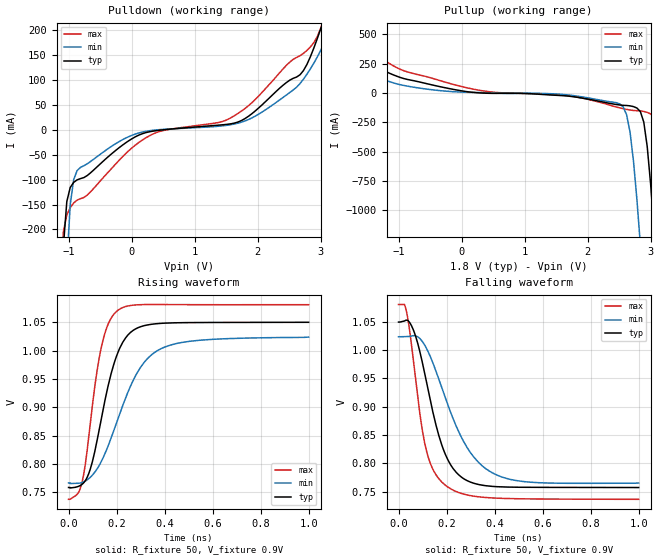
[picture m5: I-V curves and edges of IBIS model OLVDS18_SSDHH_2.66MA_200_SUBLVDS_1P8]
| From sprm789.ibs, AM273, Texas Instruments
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|   Model Cell OLVDS18_SSDHH_2.66MA_200_SUBLVDS_1P8
|OLVDS18_SSDHH_2.66MA_200_SUBLVDS_1P8
[Model]   OLVDS18_SSDHH_2.66MA_200_SUBLVDS_1P8
Model_type   Output
Polarity   Non-Inverting
Cref =  15.0001pF
Rref =  101.0000M
Vref =  0V
Vmeas =  1.08
C_comp   1.5p   1.5p   1.5p
[Temperature Range]   25   125   -40
[Voltage Range]   1.8   1.62   1.98
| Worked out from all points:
|   slope of the pulldown table from 0 to 0.27 V, typ, clamps not added: 19.7 ohm
|   slope of the pullup table from 0 to 0.27 V, typ, clamps not added: 16.2 ohm
|   rising waveform, R_fixture 50, V_fixture 0.9V: 20-80 % time 94.5ps typ, 152ps min, 67.8ps max; typ from 0.758 V to 1.05 V
|   falling waveform, R_fixture 50, V_fixture 0.9V: 20-80 % time 103ps typ, 155ps min, 74.8ps max; typ from 1.05 V to 0.757 V
| Nom Voltages:
|   BIAS1=1.2, BIAS2=1.2, VDD=1.1, VDDS=1.8, BUS_BIAS3=0, BUS_VSSS=0,
|   ESD_BIASFET=0, VSS=0
| Min Voltages:
|   BIAS1=1.2, BIAS2=1.2, VDD=0.99, VDDS=1.62, BUS_BIAS3=0, BUS_VSSS=0,
|   ESD_BIASFET=0, VSS=0
| Max Voltages:
|   BIAS1=1.2, BIAS2=1.2, VDD=1.21, VDDS=1.98, BUS_BIAS3=0, BUS_VSSS=0,
|   ESD_BIASFET=0, VSS=0
[Pulldown]
|   voltage   I(typ)   I(min)   I(max)
-1.8V     -5.997A    -6.311A    -5.864A
-1.091V   -234.2mA   -488.7mA   -204.3mA
-1.036V   -143.9mA   -270.2mA   -171mA
-927.3mV  -105.6mA   -100mA     -146.9mA
-872.7mV  -100.6mA   -82.01mA   -141.2mA
-218.2mV  -37.37mA   -24.79mA   -63.17mA
327.3mV   -2.962mA   -1.166mA   -8.921mA
1.909V    32.39mA    23.84mA    54.57mA
2.727V    118.8mA    101.5mA    153.3mA
3V        202mA      158.9mA    202.9mA
3.109V    243.4mA    214.1mA    248.6mA
3.6V      459.6mA    832.2mA    511.7mA
[Pullup]
|   voltage   I(typ)   I(min)   I(max)
-1.8V     398mA      361.1mA    551.2mA
-1.418V   248.9mA    148.1mA    355.3mA
-872.7mV  115.1mA    58.08mA    179.6mA
2.509V    -102.9mA   -93.66mA   -127.4mA
2.673V    -110.2mA   -333.6mA   -145.7mA
2.782V    -128.5mA   -906.1mA   -151.4mA
2.836V    -158.3mA   -1.288A    -153.1mA
2.945V    -454.7mA   -2.149A    -165.6mA
3.055V    -1.167A    -3.082A    -203.1mA
3.164V    -2.058A    -4.046A    -493.8mA
3.273V    -3.02A     -5.011A    -1.258A
3.6V      -6A        -7.905A    -4.194A
[Ramp]
| variable   typ   min   max
dV/dt_f 0.10272488/0.11435077n 87.218217m/0.15261476n 0.13058394/0.14245464n
dV/dt_r 0.12749001/96.124483p 90.404119m/0.14999312n 0.18248483/69.340186p
R_load = 50
[Rising Waveform]
R_fixture = 50
V_fixture = 0.9V
V_fixture_min = 0.9V
V_fixture_max = 0.9V
|   time   V(typ)   V(min)   V(max)
0s        758.3mV    766.3mV    737.3mV
52.18ps   762.5mV    766.5mV    760.9mV
87.03ps   786.1mV    774.9mV    857.9mV
114.4ps   832mV      788.2mV    952.1mV
137.9ps   882.9mV    805.4mV    1.009V
200.3ps   990.9mV    873mV      1.07V
246.2ps   1.027V     925.5mV    1.079V
295.7ps   1.042V     968.1mV    1.081V
399.4ps   1.049V     1.006V     1.082V
1ns       1.05V      1.024V     1.081V
[Falling Waveform]
R_fixture = 50
V_fixture = 0.9V
V_fixture_min = 0.9V
V_fixture_max = 0.9V
|   time   V(typ)   V(min)   V(max)
0s        1.05V      1.024V     1.081V
24.6ps    1.051V     1.024V     1.081V
36.32ps   1.053V     1.024V     1.061V
72.02ps   1.023V     1.025V     944.7mV
94.26ps   987.6mV    1.018V     871.7mV
117.5ps   941.3mV    1.002V     820.2mV
191ps     820.1mV    920.5mV    762.8mV
285.9ps   769.4mV    827.8mV    744.1mV
404.4ps   758.9mV    780.3mV    738.6mV
1ns       757.3mV    765.3mV    736.5mV
